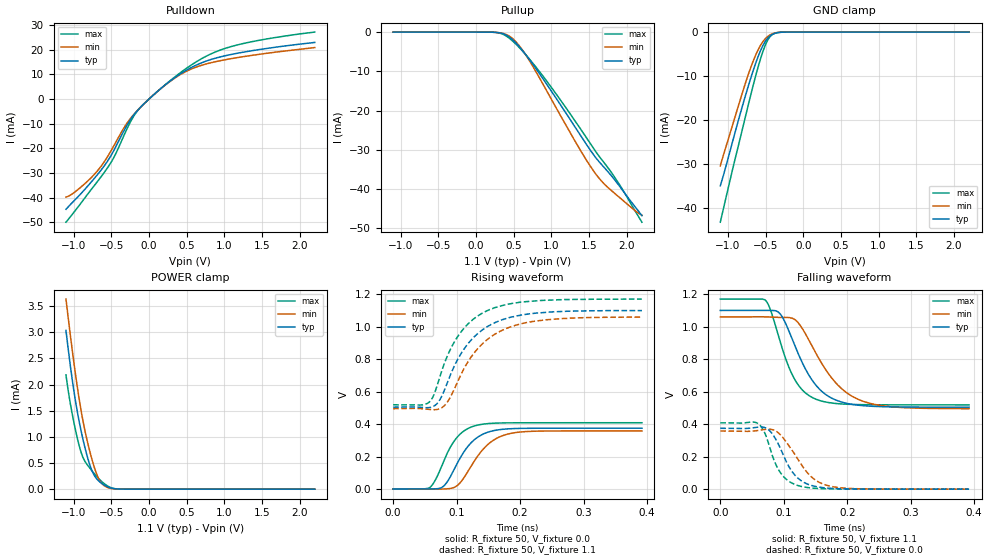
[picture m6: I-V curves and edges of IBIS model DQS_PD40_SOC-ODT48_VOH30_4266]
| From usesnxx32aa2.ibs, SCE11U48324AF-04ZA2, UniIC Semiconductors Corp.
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| DQS_PD40_SOC-ODT48_VOH30_4266
| (40 Ohm Pulldown, 48 Ohm System ODT Setting, VOH=VDDQ/3.0, 3200-4266Mbps)
[Model]   DQS_PD40_SOC-ODT48_VOH30_4266
Model_type   I/O
Vinl = 123.333mV
Vinh = 243.333mV
Vmeas = 183.333mV
Vref = 0.0mV
Cref = 0.0pF
Rref = 48.000Ohm
|   typ   min   max
|C_comp   0.838pF   0.788pF   0.888pF
C_comp_pullup   0.4190pF   0.3940pF   0.4440pF
C_comp_pulldown   0.4190pF   0.3940pF   0.4440pF
| Note: C_comp changes when the ODT circuit is enabled.
[Model Spec]
| Input threshold voltage corners
Vinl   0.1233V   0.1167V   0.1350V
Vinh   0.2433V   0.2367V   0.2550V
| Measurement voltage corners
Vmeas   0.1833V   0.1767V   0.1950V
| Timing spec test load voltage corners
Vref   0.0000V   0.0000V   0.0000V
| Dynamic Overshoot Parameters from LPDDR4 Specification
D_overshoot_ampl_h   0.30   NA   NA
D_overshoot_ampl_l   0.30   NA   NA
D_overshoot_area_h   0.1n   NA   NA
D_overshoot_area_l   0.1n   NA   NA
[Receiver Thresholds]
Vcross_low   = 123.3mV
Vcross_high  = 243.3mV
Vdiff_ac   = 120mV
Vdiff_dc   = 120mV
Tdiffslew_ac = 10.000ns |Not specified, so set to high value
[Voltage Range]   1.1000V   1.0600V   1.1700V
[Pullup Reference]   1.1000V   1.0600V   1.1700V
| Junction Temperature (Ambient temp is 35C typ 95C min -40C max)
[Temperature Range]   50.0   110.0   -40.0
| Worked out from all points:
|   slope of the pulldown table from 0 to 0.165 V, typ, clamps not added: 36.9 ohm
|   slope of the pullup table from 0 to 0.165 V, typ, clamps not added: 15.6 kohm
|   GND clamp passes 1 mA (typ) near -0.45 V on its own axis
|   POWER clamp passes 1 mA (typ) near -0.88 V on its own axis
|   rising waveform, R_fixture 50, V_fixture 0.0: 20-80 % time 36.8ps typ, 41ps min, 32.6ps max; typ from 0 V to 0.375 V
|   falling waveform, R_fixture 50, V_fixture 1.1: 20-80 % time 47ps typ, 58.8ps min, 37.1ps max; typ from 1.1 V to 0.505 V
|   rising waveform, R_fixture 50, V_fixture 1.1: 20-80 % time 58.4ps typ, 61.8ps min, 54.2ps max; typ from 0.505 V to 1.1 V
|   falling waveform, R_fixture 50, V_fixture 0.0: 20-80 % time 31.8ps typ, 40.1ps min, 26.5ps max; typ from 0.375 V to 0.001 V
[Pulldown]
|   Voltage   I(typ)   I(min)   I(max)
-1.1V     -44.75mA   -39.77mA   -50mA
-902mV    -38.42mA   -35.75mA   -42.29mA
-671mV    -30.26mA   -28.72mA   -33.02mA
-482.9mV  -21.87mA   -19.96mA   -24.7mA
-278.3mV  -9.972mA   -9.272mA   -11.31mA
-156.2mV  -4.822mA   -4.735mA   -4.963mA
137.5mV   3.741mA    3.714mA    3.748mA
375.1mV   9.367mA    9.149mA    9.729mA
695.2mV   14.68mA    13.69mA    16.33mA
1.035V    17.75mA    16.11mA    20.81mA
1.458V    20.08mA    18.15mA    23.85mA
2.2V      23.01mA    20.92mA    27.21mA
[GND Clamp]
|   Voltage   I(typ)   I(min)   I(max)
-1.1V     -34.88mA   -30.35mA   -43.13mA
-1.047V   -31.79mA   -27.25mA   -39.23mA
-941.6mV  -25.13mA   -21.34mA   -31.48mA
-789.8mV  -15.79mA   -12.83mA   -20.82mA
-667.7mV  -8.939mA   -6.742mA   -12.34mA
-595.1mV  -5.415mA   -3.908mA   -7.721mA
-525.8mV  -2.776mA   -1.982mA   -3.978mA
-473mV    -1.427mA   -1.034mA   -1.891mA
-416.9mV  -602.3uA   -443.1uA   -664.2uA
-350.9mV  -167uA     -127uA     -146.8uA
-235.4mV  -8.314uA   -7.865uA   -4.406uA
2.2V      0A         0A         0A
[Pullup]
|   Voltage   I(typ)   I(min)   I(max)
-1.1V     5.237uA    8.07uA     2.361uA
229.9mV   -37.74uA   -38.67uA   -38.87uA
345.4mV   -338.1uA   -276.7uA   -463.3uA
441.1mV   -1.249mA   -1.027mA   -1.564mA
556.6mV   -3.33mA    -3.082mA   -3.598mA
698.5mV   -6.745mA   -6.992mA   -6.645mA
975.7mV   -14.36mA   -16.29mA   -13.47mA
1.302V    -23.86mA   -27.41mA   -22.33mA
1.599V    -32.26mA   -36.44mA   -30.76mA
1.718V    -34.88mA   -39.02mA   -33.75mA
1.89V     -38.9mA    -41.91mA   -38.47mA
2.2V      -46.77mA   -46.64mA   -48.43mA
[POWER Clamp]
|   Voltage   I(typ)   I(min)   I(max)
-1.1V     3.036mA    3.636mA    2.186mA
-1.041V   2.347mA    2.931mA    1.626mA
-977.9mV  1.724mA    2.242mA    1.161mA
-911.9mV  1.201mA    1.612mA    764.9uA
-859.1mV  857.7uA    1.196mA    561.5uA
-799.7mV  537uA      814.2uA    433.5uA
-740.3mV  306uA      494.6uA    324.3uA
-667.7mV  159.9uA    206.1uA    205.2uA
-598.4mV  83.69uA    71.98uA    113.1uA
-489.5mV  17.77uA    10.88uA    22.46uA
-367.4mV  1.206uA    882.7nA    945.9nA
2.2V      0A         0A         0A
[Ramp]
|   typ   min   max
| 20% - 80%
dV/dt_r   224.64m/36.81p   214.61m/40.96p   244.92m/32.64p
dV/dt_f   357.19m/47.02p   338.70m/58.80p   390.62m/37.08p
| 25% - 75%
|dV/dt_r   187.20m/29.36p   178.84m/32.70p   204.10m/25.93p
|dV/dt_f   297.66m/37.50p   282.25m/46.95p   325.51m/29.52p
R_load = 50
[Rising Waveform]
R_fixture = 50
V_fixture = 0.0
|   Time   V(typ)   V(min)   V(max)
0s        456.8uV    388.7uV    331.3uV
57ps      217uV      98.01uV    8.005mV
67ps      1.673mV    -468.4uV   59.29mV
77ps      10.79mV    240.9uV    147.4mV
101ps     158.5mV    21.74mV    320mV
116ps     253.8mV    96.97mV    368.9mV
131ps     313.3mV    190.7mV    392.1mV
157ps     358.8mV    298.3mV    405.4mV
189ps     372.5mV    345.6mV    408.2mV
392ps     374.9mV    358.1mV    408.5mV
[Falling Waveform]
R_fixture   = 50
V_fixture   = 1.1
V_fixture_min = 1.06
V_fixture_max = 1.17
|   Time   V(typ)   V(min)   V(max)
0s        1.1V       1.06V      1.17V
72ps      1.1V       1.06V      1.159V
80ps      1.1V       1.059V     1.093V
95ps      1.076V     1.057V     899.3mV
114ps     916.7mV    1.051V     699.3mV
131ps     764mV      977.7mV    603.7mV
151ps     638.5mV    834.2mV    553.4mV
185ps     544.4mV    641.8mV    526.4mV
223ps     514.7mV    544mV      520.3mV
392ps     504.7mV    495.5mV    519mV
[Rising Waveform]
R_fixture   = 50
V_fixture   = 1.1
V_fixture_min = 1.06
V_fixture_max = 1.17
|   Time   V(typ)   V(min)   V(max)
0s        504.5mV    495.1mV    518.9mV
56ps      501.5mV    490.7mV    532.7mV
65ps      512.8mV    488.6mV    588mV
78ps      583.3mV    504.7mV    744.4mV
93ps      728.3mV    587.7mV    882mV
112ps     863.8mV    744.1mV    991.8mV
132ps     953mV      859.1mV    1.062V
155ps     1.015V     940.2mV    1.11V
227ps     1.084V     1.036V     1.16V
392ps     1.099V     1.059V     1.17V
[Falling Waveform]
R_fixture = 50
V_fixture = 0.0
|   Time   V(typ)   V(min)   V(max)
0s        375mV      358.2mV    408.6mV
57ps      381.3mV    360mV      409.2mV
74ps      371.9mV    369.3mV    306.6mV
85ps      323mV      362.9mV    175.1mV
95ps      248.6mV    333.9mV    100.3mV
109ps     133mV      262.6mV    46.49mV
124ps     62.5mV     174.5mV    20.74mV
148ps     18.69mV    61.64mV    6.015mV
178ps     4.653mV    14.94mV    1.552mV
392ps     521.4uV    478.9uV    359.4uV
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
